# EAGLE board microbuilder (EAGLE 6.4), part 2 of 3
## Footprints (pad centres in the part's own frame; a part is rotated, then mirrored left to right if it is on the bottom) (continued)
LOWPASSFILTER0603 = smd 0.2 x 0.6: P$1 0.5,0.55; P$2 0,0.55; P$3 -0.5,0.55; P$4 -0.5,-0.55; P$5 0,-0.55; P$6 0.5,-0.55
LQFP48 = smd 1.5 x 0.25: 1 -4.3,2.75; 2 -4.3,2.25; 3 -4.3,1.75; 4 -4.3,1.25; 5 -4.3,0.75; 6 -4.3,0.25; 7 -4.3,-0.25; 8 -4.3,-0.75; 9 -4.3,-1.25; 10 -4.3,-1.75; 11 -4.3,-2.25; 12 -4.3,-2.75; 25 4.3,-2.75; 26 4.3,-2.25; 27 4.3,-1.75; 28 4.3,-1.25; 29 4.3,-0.75; 30 4.3,-0.25; 31 4.3,0.25; 32 4.3,0.75; 33 4.3,1.25; 34 4.3,1.75; 35 4.3,2.25; 36 4.3,2.75 | smd 0.25 x 1.5: 13 -2.75,-4.3; 14 -2.25,-4.3; 15 -1.75,-4.3; 16 -1.25,-4.3; 17 -0.75,-4.3; 18 -0.25,-4.3; 19 0.25,-4.3; 20 0.75,-4.3; 21 1.25,-4.3; 22 1.75,-4.3; 23 2.25,-4.3; 24 2.75,-4.3; 37 2.75,4.3; 38 2.25,4.3; 39 1.75,4.3; 40 1.25,4.3; 41 0.75,4.3; 42 0.25,4.3; 43 -0.25,4.3; 44 -0.75,4.3; 45 -1.25,4.3; 46 -1.75,4.3; 47 -2.25,4.3; 48 -2.75,4.3
LQFP64 = smd 1.55 x 0.25: 1 -5.7,3.75; 2 -5.7,3.25; 3 -5.7,2.75; 4 -5.7,2.25; 5 -5.7,1.75; 6 -5.7,1.25; 7 -5.7,0.75; 8 -5.7,0.25; 9 -5.7,-0.25; 10 -5.7,-0.75; 11 -5.7,-1.25; 12 -5.7,-1.75; 13 -5.7,-2.25; 14 -5.7,-2.75; 15 -5.7,-3.25; 16 -5.7,-3.75; 33 5.7,-3.75; 34 5.7,-3.25; 35 5.7,-2.75; 36 5.7,-2.25; 37 5.7,-1.75; 38 5.7,-1.25; 39 5.7,-0.75; 40 5.7,-0.25; 41 5.7,0.25; 42 5.7,0.75; 43 5.7,1.25; 44 5.7,1.75; 45 5.7,2.25; 46 5.7,2.75; 47 5.7,3.25; 48 5.7,3.75 | smd 0.25 x 1.55: 17 -3.75,-5.7; 18 -3.25,-5.7; 19 -2.75,-5.7; 20 -2.25,-5.7; 21 -1.75,-5.7; 22 -1.25,-5.7; 23 -0.75,-5.7; 24 -0.25,-5.7; 25 0.25,-5.7; 26 0.75,-5.7; 27 1.25,-5.7; 28 1.75,-5.7; 29 2.25,-5.7; 30 2.75,-5.7; 31 3.25,-5.7; 32 3.75,-5.7; 49 3.75,5.7; 50 3.25,5.7; 51 2.75,5.7; 52 2.25,5.7; 53 1.75,5.7; 54 1.25,5.7; 55 0.75,5.7; 56 0.25,5.7; 57 -0.25,5.7; 58 -0.75,5.7; 59 -1.25,5.7; 60 -1.75,5.7; 61 -2.25,5.7; 62 -2.75,5.7; 63 -3.25,5.7; 64 -3.75,5.7
LQFP80 = smd 1.2 x 0.254: 1 -6.725,4.75; 2 -6.725,4.25; 3 -6.725,3.75; 4 -6.725,3.25; 5 -6.725,2.75; 6 -6.725,2.25; 7 -6.725,1.75; 8 -6.725,1.25; 9 -6.725,0.75; 10 -6.725,0.25; 11 -6.725,-0.25; 12 -6.725,-0.75; 13 -6.725,-1.25; 14 -6.725,-1.75; 15 -6.725,-2.25; 16 -6.725,-2.75; 17 -6.725,-3.25; 18 -6.725,-3.75; 19 -6.725,-4.25; 20 -6.725,-4.75; 41 6.725,-4.75; 42 6.725,-4.25; 43 6.725,-3.75; 44 6.725,-3.25; 45 6.725,-2.75; 46 6.725,-2.25; 47 6.725,-1.75; 48 6.725,-1.25; 49 6.725,-0.75; 50 6.725,-0.25; 51 6.725,0.25; 52 6.725,0.75; 53 6.725,1.25; 54 6.725,1.75; 55 6.725,2.25; 56 6.725,2.75; 57 6.725,3.25; 58 6.725,3.75; 59 6.725,4.25; 60 6.725,4.75 | smd 0.254 x 1.2: 21 -4.75,-6.725; 22 -4.25,-6.725; 23 -3.75,-6.725; 24 -3.25,-6.725; 25 -2.75,-6.725; 26 -2.25,-6.725; 27 -1.75,-6.725; 28 -1.25,-6.725; 29 -0.75,-6.725; 30 -0.25,-6.725; 31 0.25,-6.725; 32 0.75,-6.725; 33 1.25,-6.725; 34 1.75,-6.725; 35 2.25,-6.725; 36 2.75,-6.725; 37 3.25,-6.725; 38 3.75,-6.725; 39 4.25,-6.725; 40 4.75,-6.725; 61 4.75,6.725; 62 4.25,6.725; 63 3.75,6.725; 64 3.25,6.725; 65 2.75,6.725; 66 2.25,6.725; 67 1.75,6.725; 68 1.25,6.725; 69 0.75,6.725; 70 0.25,6.725; 71 -0.25,6.725; 72 -0.75,6.725; 73 -1.25,6.725; 74 -1.75,6.725; 75 -2.25,6.725; 76 -2.75,6.725; 77 -3.25,6.725; 78 -3.75,6.725; 79 -4.25,6.725; 80 -4.75,6.725
LQFP100 = smd 0.27 x 1.5: 1 -6,-7.75; 2 -5.5,-7.75; 3 -5,-7.75; 4 -4.5,-7.75; 5 -4,-7.75; 6 -3.5,-7.75; 7 -3,-7.75; 8 -2.5,-7.75; 9 -2,-7.75; 10 -1.5,-7.75; 11 -1,-7.75; 12 -0.5,-7.75; 13 0,-7.75; 14 0.5,-7.75; 15 1,-7.75; 16 1.5,-7.75; 17 2,-7.75; 18 2.5,-7.75; 19 3,-7.75; 20 3.5,-7.75; 21 4,-7.75; 22 4.5,-7.75; 23 5,-7.75; 24 5.5,-7.75; 25 6,-7.75; 51 6,7.75; 52 5.5,7.75; 53 5,7.75; 54 4.5,7.75; 55 4,7.75; 56 3.5,7.75; 57 3,7.75; 58 2.5,7.75; 59 2,7.75; 60 1.5,7.75; 61 1,7.75; 62 0.5,7.75; 63 0,7.75; 64 -0.5,7.75; 65 -1,7.75; 66 -1.5,7.75; 67 -2,7.75; 68 -2.5,7.75; 69 -3,7.75; 70 -3.5,7.75; 71 -4,7.75; 72 -4.5,7.75; 73 -5,7.75; 74 -5.5,7.75; 75 -6,7.75 | smd 1.5 x 0.27: 26 7.75,-6; 27 7.75,-5.5; 28 7.75,-5; 29 7.75,-4.5; 30 7.75,-4; 31 7.75,-3.5; 32 7.75,-3; 33 7.75,-2.5; 34 7.75,-2; 35 7.75,-1.5; 36 7.75,-1; 37 7.75,-0.5; 38 7.75,0; 39 7.75,0.5; 40 7.75,1; 41 7.75,1.5; 42 7.75,2; 43 7.75,2.5; 44 7.75,3; 45 7.75,3.5; 46 7.75,4; 47 7.75,4.5; 48 7.75,5; 49 7.75,5.5; 50 7.75,6; 76 -7.75,6; 77 -7.75,5.5; 78 -7.75,5; 79 -7.75,4.5; 80 -7.75,4; 81 -7.75,3.5; 82 -7.75,3; 83 -7.75,2.5; 84 -7.75,2; 85 -7.75,1.5; 86 -7.75,1; 87 -7.75,0.5; 88 -7.75,0; 89 -7.75,-0.5; 90 -7.75,-1; 91 -7.75,-1.5; 92 -7.75,-2; 93 -7.75,-2.5; 94 -7.75,-3; 95 -7.75,-3.5; 96 -7.75,-4; 97 -7.75,-4.5; 98 -7.75,-5; 99 -7.75,-5.5; 100 -7.75,-6
LQFP144 = smd 0.27 x 1.5: 1 -8.75,-10.75; 2 -8.25,-10.75; 3 -7.75,-10.75; 4 -7.25,-10.75; 5 -6.75,-10.75; 6 -6.25,-10.75; 7 -5.75,-10.75; 8 -5.25,-10.75; 9 -4.75,-10.75; 10 -4.25,-10.75; 11 -3.75,-10.75; 12 -3.25,-10.75; 13 -2.75,-10.75; 14 -2.25,-10.75; 15 -1.75,-10.75; 16 -1.25,-10.75; 17 -0.75,-10.75; 18 -0.25,-10.75; 19 0.25,-10.75; 20 0.75,-10.75; 21 1.25,-10.75; 22 1.75,-10.75; 23 2.25,-10.75; 24 2.75,-10.75; 25 3.25,-10.75; 26 3.75,-10.75; 27 4.25,-10.75; 28 4.75,-10.75; 29 5.25,-10.75; 30 5.75,-10.75; 31 6.25,-10.75; 32 6.75,-10.75; 33 7.25,-10.75; 34 7.75,-10.75; 35 8.25,-10.75; 36 8.75,-10.75; 73 8.75,10.75; 74 8.25,10.75; 75 7.75,10.75; 76 7.25,10.75; 77 6.75,10.75; 78 6.25,10.75; 79 5.75,10.75; 80 5.25,10.75; 81 4.75,10.75; 82 4.25,10.75; 83 3.75,10.75; 84 3.25,10.75; 85 2.75,10.75; 86 2.25,10.75; 87 1.75,10.75; 88 1.25,10.75; 89 0.75,10.75; 90 0.25,10.75; 91 -0.25,10.75; 92 -0.75,10.75; 93 -1.25,10.75; 94 -1.75,10.75; 95 -2.25,10.75; 96 -2.75,10.75; 97 -3.25,10.75; 98 -3.75,10.75; 99 -4.25,10.75; 100 -4.75,10.75; 101 -5.25,10.75; 102 -5.75,10.75; 103 -6.25,10.75; 104 -6.75,10.75; 105 -7.25,10.75; 106 -7.75,10.75; 107 -8.25,10.75; 108 -8.75,10.75 | smd 1.5 x 0.27: 37 10.75,-8.75; 38 10.75,-8.25; 39 10.75,-7.75; 40 10.75,-7.25; 41 10.75,-6.75; 42 10.75,-6.25; 43 10.75,-5.75; 44 10.75,-5.25; 45 10.75,-4.75; 46 10.75,-4.25; 47 10.75,-3.75; 48 10.75,-3.25; 49 10.75,-2.75; 50 10.75,-2.25; 51 10.75,-1.75; 52 10.75,-1.25; 53 10.75,-0.75; 54 10.75,-0.25; 55 10.75,0.25; 56 10.75,0.75; 57 10.75,1.25; 58 10.75,1.75; 59 10.75,2.25; 60 10.75,2.75; 61 10.75,3.25; 62 10.75,3.75; 63 10.75,4.25; 64 10.75,4.75; 65 10.75,5.25; 66 10.75,5.75; 67 10.75,6.25; 68 10.75,6.75; 69 10.75,7.25; 70 10.75,7.75; 71 10.75,8.25; 72 10.75,8.75; 109 -10.75,8.75; 110 -10.75,8.25; 111 -10.75,7.75; 112 -10.75,7.25; 113 -10.75,6.75; 114 -10.75,6.25; 115 -10.75,5.75; 116 -10.75,5.25; 117 -10.75,4.75; 118 -10.75,4.25; 119 -10.75,3.75; 120 -10.75,3.25; 121 -10.75,2.75; 122 -10.75,2.25; 123 -10.75,1.75; 124 -10.75,1.25; 125 -10.75,0.75; 126 -10.75,0.25; 127 -10.75,-0.25; 128 -10.75,-0.75; 129 -10.75,-1.25; 130 -10.75,-1.75; 131 -10.75,-2.25; 132 -10.75,-2.75; 133 -10.75,-3.25; 134 -10.75,-3.75; 135 -10.75,-4.25; 136 -10.75,-4.75; 137 -10.75,-5.25; 138 -10.75,-5.75; 139 -10.75,-6.25; 140 -10.75,-6.75; 141 -10.75,-7.25; 142 -10.75,-7.75; 143 -10.75,-8.25; 144 -10.75,-8.75
LQFP208 = smd 1.4 x 0.29: 1 -15.3,12.75; 2 -15.3,12.25; 3 -15.3,11.75; 4 -15.3,11.25; 5 -15.3,10.75; 6 -15.3,10.25; 7 -15.3,9.75; 8 -15.3,9.25; 9 -15.3,8.75; 10 -15.3,8.25; 11 -15.3,7.75; 12 -15.3,7.25; 13 -15.3,6.75; 14 -15.3,6.25; 15 -15.3,5.75; 16 -15.3,5.25; 17 -15.3,4.75; 18 -15.3,4.25; 19 -15.3,3.75; 20 -15.3,3.25; 21 -15.3,2.75; 22 -15.3,2.25; 23 -15.3,1.75; 24 -15.3,1.25; 25 -15.3,0.75; 26 -15.3,0.25; 27 -15.3,-0.25; 28 -15.3,-0.75; 29 -15.3,-1.25; 30 -15.3,-1.75; 31 -15.3,-2.25; 32 -15.3,-2.75; 33 -15.3,-3.25; 34 -15.3,-3.75; 35 -15.3,-4.25; 36 -15.3,-4.75; 37 -15.3,-5.25; 38 -15.3,-5.75; 39 -15.3,-6.25; 40 -15.3,-6.75; 41 -15.3,-7.25; 42 -15.3,-7.75; 43 -15.3,-8.25; 44 -15.3,-8.75; 45 -15.3,-9.25; 46 -15.3,-9.75; 47 -15.3,-10.25; 48 -15.3,-10.75; 49 -15.3,-11.25; 50 -15.3,-11.75; 51 -15.3,-12.25; 52 -15.3,-12.75; 105 15.3,-12.75; 106 15.3,-12.25; 107 15.3,-11.75; 108 15.3,-11.25; 109 15.3,-10.75; 110 15.3,-10.25; 111 15.3,-9.75; 112 15.3,-9.25; 113 15.3,-8.75; 114 15.3,-8.25; 115 15.3,-7.75; 116 15.3,-7.25; 117 15.3,-6.75; 118 15.3,-6.25; 119 15.3,-5.75; 120 15.3,-5.25; 121 15.3,-4.75; 122 15.3,-4.25; 123 15.3,-3.75; 124 15.3,-3.25; 125 15.3,-2.75; 126 15.3,-2.25; 127 15.3,-1.75; 128 15.3,-1.25; 129 15.3,-0.75; 130 15.3,-0.25; 131 15.3,0.25; 132 15.3,0.75; 133 15.3,1.25; 134 15.3,1.75; 135 15.3,2.25; 136 15.3,2.75; 137 15.3,3.25; 138 15.3,3.75; 139 15.3,4.25; 140 15.3,4.75; 141 15.3,5.25; 142 15.3,5.75; 143 15.3,6.25; 144 15.3,6.75; 145 15.3,7.25; 146 15.3,7.75; 147 15.3,8.25; 148 15.3,8.75; 149 15.3,9.25; 150 15.3,9.75; 151 15.3,10.25; 152 15.3,10.75; 153 15.3,11.25; 154 15.3,11.75; 155 15.3,12.25; 156 15.3,12.75 | smd 0.29 x 1.4: 53 -12.75,-15.3; 54 -12.25,-15.3; 55 -11.75,-15.3; 56 -11.25,-15.3; 57 -10.75,-15.3; 58 -10.25,-15.3; 59 -9.75,-15.3; 60 -9.25,-15.3; 61 -8.75,-15.3; 62 -8.25,-15.3; 63 -7.75,-15.3; 64 -7.25,-15.3; 65 -6.75,-15.3; 66 -6.25,-15.3; 67 -5.75,-15.3; 68 -5.25,-15.3; 69 -4.75,-15.3; 70 -4.25,-15.3; 71 -3.75,-15.3; 72 -3.25,-15.3; 73 -2.75,-15.3; 74 -2.25,-15.3; 75 -1.75,-15.3; 76 -1.25,-15.3; 77 -0.75,-15.3; 78 -0.25,-15.3; 79 0.25,-15.3; 80 0.75,-15.3; 81 1.25,-15.3; 82 1.75,-15.3; 83 2.25,-15.3; 84 2.75,-15.3; 85 3.25,-15.3; 86 3.75,-15.3; 87 4.25,-15.3; 88 4.75,-15.3; 89 5.25,-15.3; 90 5.75,-15.3; 91 6.25,-15.3; 92 6.75,-15.3; 93 7.25,-15.3; 94 7.75,-15.3; 95 8.25,-15.3; 96 8.75,-15.3; 97 9.25,-15.3; 98 9.75,-15.3; 99 10.25,-15.3; 100 10.75,-15.3; 101 11.25,-15.3; 102 11.75,-15.3; 103 12.25,-15.3; 104 12.75,-15.3; 157 12.75,15.3; 158 12.25,15.3; 159 11.75,15.3; 160 11.25,15.3; 161 10.75,15.3; 162 10.25,15.3; 163 9.75,15.3; 164 9.25,15.3; 165 8.75,15.3; 166 8.25,15.3; 167 7.75,15.3; 168 7.25,15.3; 169 6.75,15.3; 170 6.25,15.3; 171 5.75,15.3; 172 5.25,15.3; 173 4.75,15.3; 174 4.25,15.3; 175 3.75,15.3; 176 3.25,15.3; 177 2.75,15.3; 178 2.25,15.3; 179 1.75,15.3; 180 1.25,15.3; 181 0.75,15.3; 182 0.25,15.3; 183 -0.25,15.3; 184 -0.75,15.3; 185 -1.25,15.3; 186 -1.75,15.3; 187 -2.25,15.3; 188 -2.75,15.3; 189 -3.25,15.3; 190 -3.75,15.3; 191 -4.25,15.3; 192 -4.75,15.3; 193 -5.25,15.3; 194 -5.75,15.3; 195 -6.25,15.3; 196 -6.75,15.3; 197 -7.25,15.3; 198 -7.75,15.3; 199 -8.25,15.3; 200 -8.75,15.3; 201 -9.25,15.3; 202 -9.75,15.3; 203 -10.25,15.3; 204 -10.75,15.3; 205 -11.25,15.3; 206 -11.75,15.3; 207 -12.25,15.3; 208 -12.75,15.3
MICROSD = smd 0.7 x 1.5: 1 9,-10.64; 2 7.9,-10.24; 3 6.8,-10.64; 4 5.7,-11.04; 5 4.6,-10.64; 6 3.5,-11.04; 7 2.4,-10.64; 8 1.3,-10.64 | smd 1.8 x 1.4: CD1 2,-0.44; CD2 8,-0.44 | smd 1.4 x 1.9: MT1 0.4,-13.54; MT2 13.6,-14.44
MINIMOLD6 = smd 0.26 x 0.65: P$1 -0.5,-0.65; P$2 0,-0.65; P$3 0.5,-0.65; P$4 0.5,0.65; P$5 0,0.65; P$6 -0.5,0.65
MOLEX20_RIGHTANGLE = smd 1 x 4: 1 11.43,0; 3 8.89,0; 5 6.35,0; 7 3.81,0; 9 1.27,0; 11 -1.27,0; 13 -3.81,0; 15 -6.35,0; 17 -8.89,0; 19 -11.43,0 | smd 1 x 4 bottom: 2 11.43,0; 4 8.89,0; 6 6.35,0; 8 3.81,0; 10 1.27,0; 12 -1.27,0; 14 -3.81,0; 16 -6.35,0; 18 -8.89,0; 20 -11.43,0
MOUNTINGHOLE_1.0_PLATED = drill 1 pad 3: P$1 0,0
MOUNTINGHOLE_2.0_PLATED = drill 2.2 pad 3: P$1 0,0
MOUNTINGHOLE_2.5_PLATED = drill 2.5 pad 3.2: P$1 0,0
MOUNTINGHOLE_2.5_PLATED_THICK = drill 2.5 pad 4: P$1 0,0
MOUNTINGHOLE_2.8 = hole 2.8: 0,0
MOUNTINGHOLE_3.0 = hole 3: 0,0
MOUNTINGHOLE_3.0_PLATED = drill 3 pad 6.452: P$1 0,0
MOUNTINGHOLE_3.0_PLATEDTHIN = drill 3 pad 3.6: P$1 0,0
MOUNTINGHOLE_3.2 = hole 3.2: 0,0
MSOP8_0.65MM = smd 0.4 x 1.4: 1 -0.975,-2.2; 2 -0.325,-2.2; 3 0.325,-2.2; 4 0.975,-2.2; 5 0.975,2.2; 6 0.325,2.2; 7 -0.325,2.2; 8 -0.975,2.2
MSOP10 = smd 0.25 x 1: 1 -1,-2.113; 2 -0.5,-2.113; 3 0,-2.113; 4 0.5,-2.113; 5 1,-2.113; 6 1,2.113; 7 0.5,2.113; 8 0,2.113; 9 -0.5,2.113; 10 -1,2.113
OSC_3.2X2.5MM = smd 1.4 x 1.2: 1 -1.1,-0.8; 2 1.1,-0.8; 3 1.1,0.8; 4 -1.1,0.8
OSC_7X5MM = smd 1.8 x 2: 1 -2.54,-2.1; 2 2.54,-2.1; 3 2.54,2.1; 4 -2.54,2.1
PAD-1.5X2.0 = smd 1.5 x 2: P$1 0,0
PANASONIC_C = smd 2.6 x 1.4: + 2.05,0; - -2.05,0
PANASONIC_D = smd 3.556 x 1.4: + 2.654,0; - -2.654,0
PSP_BACKLIGHTCON = smd 0.28 x 1.4: NC1 -0.25,0; NC2 0.25,0; VLED+ 0.75,0; VLED- -0.75,0 | smd 2.667 x 1.27: P$1 -2.54,-1.27; P$2 2.54,-1.27
PSP_TSCON = smd 0.6 x 2.3: X1 1.5,1.15; X2 -0.5,1.15; Y1 -1.5,1.15; Y2 0.5,1.15
PTC1210 = smd 1 x 3.2: P$1 -1.5,0; P$2 1.5,0
PTC1812 = smd 1.5 x 3.7: P$1 -2.1,0; P$2 2.1,0
PUSHBUTTON_SMD_SJ = smd 2 x 2: P$1 3,0; P$2 -3,0
QFN16_3MM = smd 0.8 x 0.28: P$1 -1.5,0.75; P$2 -1.5,0.25; P$3 -1.5,-0.25; P$4 -1.5,-0.75; P$9 1.5,-0.75; P$10 1.5,-0.25; P$11 1.5,0.25; P$12 1.5,0.75 | smd 0.28 x 0.8: P$5 -0.75,-1.5; P$6 -0.25,-1.5; P$7 0.25,-1.5; P$8 0.75,-1.5; P$13 0.75,1.5; P$14 0.25,1.5; P$15 -0.25,1.5; P$16 -0.75,1.5 | smd 1.5 x 1.5: THERMAL 0,0
QFN20_3MM = smd 0.7 x 0.2: 1 -1.4,0.8; 2 -1.4,0.4; 3 -1.4,0; 4 -1.4,-0.4; 5 -1.4,-0.8; 11 1.4,-0.8; 12 1.4,-0.4; 13 1.4,0; 14 1.4,0.4; 15 1.4,0.8 | smd 0.2 x 0.7: 6 -0.8,-1.4; 7 -0.4,-1.4; 8 0,-1.4; 9 0.4,-1.4; 10 0.8,-1.4; 16 0.8,1.4; 17 0.4,1.4; 18 0,1.4; 19 -0.4,1.4; 20 -0.8,1.4 | smd 1.6 x 1.6: 21 0,0
QFN20_4MM = smd 0.73 x 0.28: P$1 -1.965,1; P$2 -1.965,0.5; P$3 -1.965,0; P$4 -1.965,-0.5; P$5 -1.965,-1; P$11 1.965,-1; P$12 1.965,-0.5; P$13 1.965,0; P$14 1.965,0.5; P$15 1.965,1 | smd 0.28 x 0.73: P$6 -1,-1.965; P$7 -0.5,-1.965; P$8 0,-1.965; P$9 0.5,-1.965; P$10 1,-1.965; P$16 1,1.965; P$17 0.5,1.965; P$18 0,1.965; P$19 -0.5,1.965; P$20 -1,1.965 | smd 2.5 x 2.5: P$21 0,0
QFN24_4MM = smd 0.8 x 0.28: 1 -2,1.25; 2 -2,0.75; 3 -2,0.25; 4 -2,-0.25; 5 -2,-0.75; 6 -2,-1.25; 13 2,-1.25; 14 2,-0.75; 15 2,-0.25; 16 2,0.25; 17 2,0.75; 18 2,1.25 | smd 0.28 x 0.8: 7 -1.25,-2; 8 -0.75,-2; 9 -0.25,-2; 10 0.25,-2; 11 0.75,-2; 12 1.25,-2; 19 1.25,2; 20 0.75,2; 21 0.25,2; 22 -0.25,2; 23 -0.75,2; 24 -1.25,2 | smd 1.778 x 1.778: THERM 0,0
QFN28_5MM = smd 1.15 x 0.27: 1 -2.4,1.5; 2 -2.4,1; 3 -2.4,0.5; 4 -2.4,0; 5 -2.4,-0.5; 6 -2.4,-1; 7 -2.4,-1.5; 15 2.4,-1.5; 16 2.4,-1; 17 2.4,-0.5; 18 2.4,0; 19 2.4,0.5; 20 2.4,1; 21 2.4,1.5 | smd 0.27 x 1.15: 8 -1.5,-2.4; 9 -1,-2.4; 10 -0.5,-2.4; 11 0,-2.4; 12 0.5,-2.4; 13 1,-2.4; 14 1.5,-2.4; 22 1.5,2.4; 23 1,2.4; 24 0.5,2.4; 25 0,2.4; 26 -0.5,2.4; 27 -1,2.4; 28 -1.5,2.4 | smd 3.15 x 3.15: THERMAL 0,0
QFN32_5MM = smd 0.8 x 0.25: 1 -2.5,1.75; 2 -2.5,1.25; 3 -2.5,0.75; 4 -2.5,0.25; 5 -2.5,-0.25; 6 -2.5,-0.75; 7 -2.5,-1.25; 8 -2.5,-1.75; 17 2.5,-1.75; 18 2.5,-1.25; 19 2.5,-0.75; 20 2.5,-0.25; 21 2.5,0.25; 22 2.5,0.75; 23 2.5,1.25; 24 2.5,1.75 | smd 0.25 x 0.8: 9 -1.75,-2.5; 10 -1.25,-2.5; 11 -0.75,-2.5; 12 -0.25,-2.5; 13 0.25,-2.5; 14 0.75,-2.5; 15 1.25,-2.5; 16 1.75,-2.5; 25 1.75,2.5; 26 1.25,2.5; 27 0.75,2.5; 28 0.25,2.5; 29 -0.25,2.5; 30 -0.75,2.5; 31 -1.25,2.5; 32 -1.75,2.5 | smd 3.5 x 3.5: 33 0,0
QSOP24_0.635MM = smd 0.3 x 1.7: 1 -3.493,-2.935; 2 -2.857,-2.935; 3 -2.223,-2.935; 4 -1.587,-2.935; 5 -0.953,-2.935; 6 -0.318,-2.935; 7 0.318,-2.935; 8 0.953,-2.935; 9 1.587,-2.935; 10 2.223,-2.935; 11 2.857,-2.935; 12 3.493,-2.935; 13 3.493,2.935; 14 2.857,2.935; 15 2.223,2.935; 16 1.587,2.935; 17 0.953,2.935; 18 0.318,2.935; 19 -0.318,2.935; 20 -0.953,2.935; 21 -1.587,2.935; 22 -2.223,2.935; 23 -2.857,2.935; 24 -3.493,2.935
RASBERRYPI_IDC = drill 1 pad 1.676 square: 1 -1.27,15.24 | drill 1 pad 1.676: 2 1.27,15.24; 3 -1.27,12.7; 4 1.27,12.7; 5 -1.27,10.16; 6 1.27,10.16; 7 -1.27,7.62; 8 1.27,7.62; 9 -1.27,5.08; 10 1.27,5.08; 11 -1.27,2.54; 12 1.27,2.54; 13 -1.27,0; 14 1.27,0; 15 -1.27,-2.54; 16 1.27,-2.54; 17 -1.27,-5.08; 18 1.27,-5.08; 19 -1.27,-7.62; 20 1.27,-7.62; 21 -1.27,-10.16; 22 1.27,-10.16; 23 -1.27,-12.7; 24 1.27,-12.7; 25 -1.27,-15.24; 26 1.27,-15.24
RASBERRYPI_SHIELD = drill 1 pad 1.676 square: 1 51.308,82.55 | drill 1 pad 1.676: 2 53.848,82.55; 3 51.308,80.01; 4 53.848,80.01; 5 51.308,77.47; 6 53.848,77.47; 7 51.308,74.93; 8 53.848,74.93; 9 51.308,72.39; 10 53.848,72.39; 11 51.308,69.85; 12 53.848,69.85; 13 51.308,67.31; 14 53.848,67.31; 15 51.308,64.77; 16 53.848,64.77; 17 51.308,62.23; 18 53.848,62.23; 19 51.308,59.69; 20 53.848,59.69; 21 51.308,57.15; 22 53.848,57.15; 23 51.308,54.61; 24 53.848,54.61; 25 51.308,52.07; 26 53.848,52.07
RESPACK_4X0603 = smd 0.65 x 0.8: 1 -1.3,-0.75; 4 1.3,-0.75; 5 1.3,0.75; 8 -1.3,0.75 | smd 0.5 x 0.8: 2 -0.4,-0.75; 3 0.4,-0.75; 6 0.4,0.75; 7 -0.4,0.75
RGBLED_PLCC4 = smd 1.1 x 1: 1 -1.4,0.6; 2 -1.4,-0.6; 3 1.4,-0.6; 4 1.4,0.6
RGBLED_PLCC6 = smd 1 x 2: 1 -1.6,-2.158; 2 0,-2.158; 3 1.6,-2.158; 4 1.6,2.108; 5 0,2.108; 6 -1.6,2.108
RJ45PTH = drill 0.9: 1 3.57,2.54; 2 2.55,4.32; 3 1.53,2.54; 4 0.51,4.32; 5 -0.51,2.54; 6 -1.53,4.32; 7 -2.55,2.54; 8 -3.57,4.32; 9 -6.86,9.18; 10 -4.57,9.18; 11 4.57,9.18; 12 6.86,9.18 | drill 1.6: P$11 -8.13,3.43; P$12 8.13,3.43 | hole 3.2: -6.35,0; 6.35,0
RJ45SMT = smd 0.61 x 3.05: 1 3.57,9.98; 2 2.55,9.98; 3 1.53,9.98; 4 0.51,9.98; 5 -0.51,9.98; 6 -1.53,9.98; 7 -2.55,9.98; 8 -3.57,9.98; 9 -6.975,10.8; 10 -5.705,10.8; 11 5.705,10.8; 12 6.975,10.8 | smd 2 x 3.05: P$13 8.66,0; P$14 -8.89,0 | hole 3.25: -6.35,0; 6.35,0
RJ45_PULSEJACK = drill 0.9: 1 4.445,-6.35; 2 3.175,-8.89; 3 1.905,-6.35; 4 0.635,-8.89; 5 -0.635,-6.35; 6 -1.905,-8.89; 7 -3.175,-6.35; 8 -4.445,-8.89 | drill 1: 9 6.325,4.9; 10 3.785,3.38; 11 -3.785,4.9; 12 -6.325,3.38 | drill 1.6: P$5 -7.875,-3.05; P$6 7.875,-3.05 | hole 3.2: -5.715,0; 5.715,0
S6B33B6_1.5IN_LCD = smd 0.5 x 3: P$1 -12.8,-6.25; P$2 -12,-6.25; P$3 -11.2,-6.25; P$4 -10.4,-6.25; P$5 -9.6,-6.25; P$6 -8.8,-6.25; P$7 -8,-6.25; P$8 -7.2,-6.25; P$9 -6.4,-6.25; P$10 -5.6,-6.25; P$11 -4.8,-6.25; P$12 -4,-6.25; P$13 -3.2,-6.25; P$14 -2.4,-6.25; P$15 -1.6,-6.25; P$16 -0.8,-6.25; P$17 0,-6.25; P$18 0.8,-6.25; P$19 1.6,-6.25; P$20 2.4,-6.25; P$21 3.2,-6.25; P$22 4,-6.25; P$23 4.8,-6.25; P$24 5.6,-6.25; P$25 6.4,-6.25; P$26 7.2,-6.25; P$27 8,-6.25; P$28 8.8,-6.25; P$29 9.6,-6.25; P$30 10.4,-6.25; P$31 11.2,-6.25; P$32 12,-6.25; P$33 12.8,-6.25 | hole 1: 12.8,-9.8; -12.8,-9.8
SC70-6L = smd 0.35 x 0.8: 1 -0.65,-0.85; 2 0,-0.85; 3 0.65,-0.85; 4 0.65,0.85; 5 0,0.85; 6 -0.65,0.85
SDCARD_PCBCARRIER_DIM = smd 1.4 x 3.4: P$1 -6.875,0; P$2 -4.375,0; P$5 3.125,0; P$6 5.625,0; P$9 -9.375,-2.3 | smd 1.4 x 3.6: P$3 -1.875,0.1; P$4 0.625,0.1 | smd 1.1 x 3.4: P$7 8.05,0 | smd 0.9 x 3.4: P$8 9.75,0
SDCARD_PCBCARRIER_DOCU = smd 1.4 x 3.4: P$1 -6.875,0; P$2 -4.375,0; P$5 3.125,0; P$6 5.625,0; P$9 -9.375,-2.3 | smd 1.4 x 3.6: P$3 -1.875,0.1; P$4 0.625,0.1 | smd 1.1 x 3.4: P$7 8.05,0 | smd 0.9 x 3.4: P$8 9.75,0
SDCARD_SMT_4U06132 = smd 1 x 2.008: 1 6.88,11.254; 2 4.38,11.254; 3 1.88,11.254; 4 -0.62,11.254; 5 -3.12,11.254; 6 -5.62,11.254; 7 -8.12,11.254; 9 9.38,11.254 | smd 0.6 x 2.008: 8 -9.845,11.254; CD -11.045,11.254; WP -12.245,11.254 | smd 1.6 x 2.8: GND -14.1,-12.35; NC1 -14.1,9.15; NC2 11.631,9.15; NC3 13.6,-12.35 | hole 1.6: 9.5,8.2 | hole 1.1: -11.5,8.2
SDCARD_SMT_4U19646 = smd 1.05 x 1.56: CD 1.02,15.47; P$1 6.77,15.47; P$2 4.27,15.47; P$3 2.52,15.47; P$4 -0.73,15.47; P$5 -3.23,15.47; P$6 -5.73,15.47; P$7 -8.15,15.47; P$8 -9.85,15.47; P$9 9.27,15.47; WP -13.2,15.47 | smd 1.2 x 2: GND@1 14.8,-5.6; GND@2 -14.8,-5.6 | hole 1.8: -12.1,-8.9; 12.1,-8.9
SEGMENT-BL-Q56C43 = drill 0.8 pad 1.778: P$1 -7.62,-7.62; P$2 -5.08,-7.62; P$3 -2.54,-7.62; P$4 0,-7.62; P$5 2.54,-7.62; P$6 5.08,-7.62; P$7 7.62,-7.62; P$8 7.62,7.62; P$9 5.08,7.62; P$10 2.54,7.62; P$11 0,7.62; P$12 -2.54,7.62; P$13 -5.08,7.62; P$14 -7.62,7.62
SEGMENT_BICOL_BL-AR12Z3010 = drill 0.8 pad 1.676: 1 -3.6,7.57; 2 -3.6,5.03; 3 -3.6,2.49; 4 -3.6,-0.05; 5 -3.6,-2.59; 6 -3.6,-5.13; 7 -3.6,-7.67; 8 3.6,-7.57; 9 3.6,-5.03; 10 3.6,-2.49; 11 3.6,0.05; 12 3.6,2.59; 13 3.6,5.13; 14 3.6,7.67
SEGMENT_BICOL_BL-M12A883XX = drill 0.8 pad 1.676: 1 -13.97,-12; 2 -11.43,-12; 3 -8.89,-12; 4 -6.35,-12; 5 -3.81,-12; 6 -1.27,-12; 7 1.27,-12; 8 3.81,-12; 9 6.35,-12; 10 8.89,-12; 11 11.43,-12; 12 13.97,-12; 13 13.97,12; 14 11.43,12; 15 8.89,12; 16 6.35,12; 17 3.81,12; 18 1.27,12; 19 -1.27,12; 20 -3.81,12; 21 -6.35,12; 22 -8.89,12; 23 -11.43,12; 24 -13.97,12
SEGMENT_BL-M07C881UR = drill 0.8 pad 1.676: 1 -8.75,-7.5; 2 -6.25,-7.5; 3 -3.75,-7.5; 4 -1.25,-7.5; 5 1.25,-7.5; 6 3.75,-7.5; 7 6.25,-7.5; 8 8.75,-7.5; 9 8.75,7.5; 10 6.25,7.5; 11 3.75,7.5; 12 1.25,7.5; 13 -1.25,7.5; 14 -3.75,7.5; 15 -6.25,7.5; 16 -8.75,7.5
SEGMENT_BL-M12A881UR = drill 0.8 pad 1.676: 1 -8.89,-12; 2 -6.35,-12; 3 -3.81,-12; 4 -1.27,-12; 5 1.27,-12; 6 3.81,-12; 7 6.35,-12; 8 8.89,-12; 9 8.89,12; 10 6.35,12; 11 3.81,12; 12 1.27,12; 13 -1.27,12; 14 -3.81,12; 15 -6.35,12; 16 -8.89,12
SEGMENT_BL-M12A883 = drill 0.8 pad 1.676: 1 -8.89,-12; 2 -6.35,-12; 3 -3.81,-12; 4 -1.27,-12; 5 1.27,-12; 6 3.81,-12; 7 6.35,-12; 8 8.89,-12; 9 8.89,12; 10 6.35,12; 11 3.81,12; 12 1.27,12; 13 -1.27,12; 14 -3.81,12; 15 -6.35,12; 16 -8.89,12
SEGMENT_BL-Q39A-42 = drill 0.8: P$1 -8.89,-5.08; P$2 -6.35,-5.08; P$3 -3.81,-5.08; P$4 -1.27,-5.08; P$5 1.27,-5.08; P$6 3.81,-5.08; P$7 6.35,-5.08; P$8 8.89,-5.08; P$9 8.89,5.08; P$10 6.35,5.08; P$11 3.81,5.08; P$12 1.27,5.08; P$13 -1.27,5.08; P$14 -3.81,5.08; P$15 -6.35,5.08; P$16 -8.89,5.08
SEGMENT_STARBURST_BL-S80A-13 = drill 0.8 pad 1.676: 1 -7.62,10.16; 2 -7.62,7.62; 3 -7.62,5.08; 4 -7.62,2.54; 5 -7.62,0; 6 -7.62,-2.54; 7 -7.62,-5.08; 8 -7.62,-7.62; 9 -7.62,-10.16; 10 7.62,-10.16; 11 7.62,-7.62; 12 7.62,-5.08; 13 7.62,-2.54; 14 7.62,0; 15 7.62,2.54; 16 7.62,5.08; 17 7.62,7.62; 18 7.62,10.16
SEGMENT_STARBURST_BL-S230B-12 = drill 0.8 pad 1.676: 1 -11.43,-30.1; 2 -8.89,-30.1; 3 -6.35,-30.1; 4 -3.81,-30.1; 5 -1.27,-30.1; 6 1.27,-30.1; 7 3.81,-30.1; 8 6.35,-30.1; 9 8.89,-30.1; 10 11.43,-30.1; 11 11.43,30.1; 12 8.89,30.1; 13 6.35,30.1; 14 3.81,30.1; 15 1.27,30.1; 16 -1.27,30.1; 17 -3.81,30.1; 18 -6.35,30.1; 19 -8.89,30.1; 20 -11.43,30.1
SI473X_SSOP = smd 1.55 x 0.35: P$1 -2.625,3.493; P$2 -2.625,2.857; P$3 -2.625,2.223; P$4 -2.625,1.587; P$5 -2.625,0.953; P$6 -2.625,0.318; P$7 -2.625,-0.318; P$8 -2.625,-0.953; P$9 -2.625,-1.587; P$10 -2.625,-2.223; P$11 -2.625,-2.857; P$12 -2.625,-3.493; P$13 2.625,-3.493; P$14 2.625,-2.857; P$15 2.625,-2.223; P$16 2.625,-1.587; P$17 2.625,-0.953; P$18 2.625,-0.318; P$19 2.625,0.318; P$20 2.625,0.953; P$21 2.625,1.587; P$22 2.625,2.223; P$23 2.625,2.857; P$24 2.625,3.493
SIM900B_SMT = smd 0.25 x 1.35: 1 -7.25,-1.475; 2 -7.25,1.475; 3 -6.75,-1.475; 4 -6.75,1.475; 5 -6.25,-1.475; 6 -6.25,1.475; 7 -5.75,-1.475; 8 -5.75,1.475; 9 -5.25,-1.475; 10 -5.25,1.475; 11 -4.75,-1.475; 12 -4.75,1.475; 13 -4.25,-1.475; 14 -4.25,1.475; 15 -3.75,-1.475; 16 -3.75,1.475; 17 -3.25,-1.475; 18 -3.25,1.475; 19 -2.75,-1.475; 20 -2.75,1.475; 21 -2.25,-1.475; 22 -2.25,1.475; 23 -1.75,-1.475; 24 -1.75,1.475; 25 -1.25,-1.475; 26 -1.25,1.475; 27 -0.75,-1.475; 28 -0.75,1.475; 29 -0.25,-1.475; 30 -0.25,1.475; 31 0.25,-1.475; 32 0.25,1.475; 33 0.75,-1.475; 34 0.75,1.475; 35 1.25,-1.475; 36 1.25,1.475; 37 1.75,-1.475; 38 1.75,1.475; 39 2.25,-1.475; 40 2.25,1.475; 41 2.75,-1.475; 42 2.75,1.475; 43 3.25,-1.475; 44 3.25,1.475; 45 3.75,-1.475; 46 3.75,1.475; 47 4.25,-1.475; 48 4.25,1.475; 49 4.75,-1.475; 50 4.75,1.475; 51 5.25,-1.475; 52 5.25,1.475; 53 5.75,-1.475; 54 5.75,1.475; 55 6.25,-1.475; 56 6.25,1.475; 57 6.75,-1.475; 58 6.75,1.475; 59 7.25,-1.475; 60 7.25,1.475 | drill 1.5 pad 2.54: P$1 -6.63,29.25; P$2 8.09,16.86; P$3 -30.89,9.41; P$4 -14.53,-2.72
SIM900_SMT = smd 2 x 0.6: P$1 -12.4,8; P$2 -12.4,7; P$3 -12.4,6; P$4 -12.4,5; P$5 -12.4,4; P$6 -12.4,3; P$7 -12.4,2; P$8 -12.4,1; P$9 -12.4,0; P$10 -12.4,-1; P$11 -12.4,-2; P$12 -12.4,-3; P$13 -12.4,-4; P$14 -12.4,-5; P$15 -12.4,-6; P$16 -12.4,-7; P$17 -12.4,-8; P$35 12.4,-8; P$36 12.4,-7; P$37 12.4,-6; P$38 12.4,-5; P$39 12.4,-4; P$40 12.4,-3; P$41 12.4,-2; P$42 12.4,-1; P$43 12.4,0; P$44 12.4,1; P$45 12.4,2; P$46 12.4,3; P$47 12.4,4; P$48 12.4,5; P$49 12.4,6; P$50 12.4,7; P$51 12.4,8 | smd 0.6 x 2: P$18 -8,-12.4; P$19 -7,-12.4; P$20 -6,-12.4; P$21 -5,-12.4; P$22 -4,-12.4; P$23 -3,-12.4; P$24 -2,-12.4; P$25 -1,-12.4; P$26 0,-12.4; P$27 1,-12.4; P$28 2,-12.4; P$29 3,-12.4; P$30 4,-12.4; P$31 5,-12.4; P$32 6,-12.4; P$33 7,-12.4; P$34 8,-12.4; P$52 8,12.4; P$53 7,12.4; P$54 6,12.4; P$55 5,12.4; P$56 4,12.4; P$57 3,12.4; P$58 2,12.4; P$59 1,12.4; P$60 0,12.4; P$61 -1,12.4; P$62 -2,12.4; P$63 -3,12.4; P$64 -4,12.4; P$65 -5,12.4; P$66 -6,12.4; P$67 -7,12.4; P$68 -8,12.4
SIM908 = smd 1.8 x 0.6: P$1 -15,9.5; P$2 -15,8.5; P$3 -15,7.5; P$4 -15,6.5; P$5 -15,5.5; P$6 -15,4.5; P$7 -15,3.5; P$8 -15,2.5; P$9 -15,1.5; P$10 -15,0.5; P$11 -15,-0.5; P$12 -15,-1.5; P$13 -15,-2.5; P$14 -15,-3.5; P$15 -15,-4.5; P$16 -15,-5.5; P$17 -15,-6.5; P$18 -15,-7.5; P$19 -15,-8.5; P$20 -15,-9.5; P$41 15,-9.5; P$42 15,-8.5; P$43 15,-7.5; P$44 15,-6.5; P$45 15,-5.5; P$46 15,-4.5; P$47 15,-3.5; P$48 15,-2.5; P$49 15,-1.5; P$50 15,-0.5; P$51 15,0.5; P$52 15,1.5; P$53 15,2.5; P$54 15,3.5; P$55 15,4.5; P$56 15,5.5; P$57 15,6.5; P$58 15,7.5; P$59 15,8.5; P$60 15,9.5 | smd 0.6 x 1.8: P$21 -9.5,-15; P$22 -8.5,-15; P$23 -7.5,-15; P$24 -6.5,-15; P$25 -5.5,-15; P$26 -4.5,-15; P$27 -3.5,-15; P$28 -2.5,-15; P$29 -1.5,-15; P$30 -0.5,-15; P$31 0.5,-15; P$32 1.5,-15; P$33 2.5,-15; P$34 3.5,-15; P$35 4.5,-15; P$36 5.5,-15; P$37 6.5,-15; P$38 7.5,-15; P$39 8.5,-15; P$40 9.5,-15; P$61 9.5,15; P$62 8.5,15; P$63 7.5,15; P$64 6.5,15; P$65 5.5,15; P$66 4.5,15; P$67 3.5,15; P$68 2.5,15; P$69 1.5,15; P$70 0.5,15; P$71 -0.5,15; P$72 -1.5,15; P$73 -2.5,15; P$74 -3.5,15; P$75 -4.5,15; P$76 -5.5,15; P$77 -6.5,15; P$78 -7.5,15; P$79 -8.5,15; P$80 -9.5,15
SIM_5002 = smd 2.54 x 1.27: 1 0.904,0.574; 2 0.904,3.114; 3 0.904,5.654; 5 26.299,0.594; 6 26.299,3.134; 7 26.299,5.674 | hole 1.7: 21.8,-1.6 | hole 1.2: 6,10.4
SMA90_DIP = drill 1.5 pad 2.54: ANTENNA 0,0 | drill 1.6 pad 2.54: GND1 -2.54,2.54; GND2 2.54,2.54; GND3 -2.54,-2.54; GND4 2.54,-2.54
SMADIODE = smd 2.54 x 2.54: A 2.349,0; C -2.349,0
SMB_DIP = drill 1.5 pad 2.54: ANTENNA 0,0 | drill 1.6 pad 2.54: GND1 -2.54,2.54; GND2 2.54,2.54; GND3 -2.54,-2.54; GND4 2.54,-2.54
SOCKET_LBGA256_8117-256-4E-01 = drill 0.43 pad 0.7 octagon: A1 7.5,7.5; A2 7.5,6.5; A3 7.5,5.5; A4 7.5,4.5; A5 7.5,3.5; A6 7.5,2.5; A7 7.5,1.5; A8 7.5,0.5; A9 7.5,-0.5; A10 7.5,-1.5; A11 7.5,-2.5; A12 7.5,-3.5; A13 7.5,-4.5; A14 7.5,-5.5; A15 7.5,-6.5; A16 7.5,-7.5; B1 6.5,7.5; B2 6.5,6.5; B3 6.5,5.5; B4 6.5,4.5; B5 6.5,3.5; B6 6.5,2.5; B7 6.5,1.5; B8 6.5,0.5; B9 6.5,-0.5; B10 6.5,-1.5; B11 6.5,-2.5; B12 6.5,-3.5; B13 6.5,-4.5; B14 6.5,-5.5; B15 6.5,-6.5; B16 6.5,-7.5; C1 5.5,7.5; C2 5.5,6.5; C3 5.5,5.5; C4 5.5,4.5; C5 5.5,3.5; C6 5.5,2.5; C7 5.5,1.5; C8 5.5,0.5; C9 5.5,-0.5; C10 5.5,-1.5; C11 5.5,-2.5; C12 5.5,-3.5; C13 5.5,-4.5; C14 5.5,-5.5; C15 5.5,-6.5; C16 5.5,-7.5; D1 4.5,7.5; D2 4.5,6.5; D3 4.5,5.5; D4 4.5,4.5; D5 4.5,3.5; D6 4.5,2.5; D7 4.5,1.5; D8 4.5,0.5; D9 4.5,-0.5; D10 4.5,-1.5; D11 4.5,-2.5; D12 4.5,-3.5; D13 4.5,-4.5; D14 4.5,-5.5; D15 4.5,-6.5; D16 4.5,-7.5; E1 3.5,7.5; E2 3.5,6.5; E3 3.5,5.5; E4 3.5,4.5; E5 3.5,3.5; E6 3.5,2.5; E7 3.5,1.5; E8 3.5,0.5; E9 3.5,-0.5; E10 3.5,-1.5; E11 3.5,-2.5; E12 3.5,-3.5; E13 3.5,-4.5; E14 3.5,-5.5; E15 3.5,-6.5; E16 3.5,-7.5; F1 2.5,7.5; F2 2.5,6.5; F3 2.5,5.5; F4 2.5,4.5; F5 2.5,3.5; F6 2.5,2.5; F7 2.5,1.5; F8 2.5,0.5; F9 2.5,-0.5; F10 2.5,-1.5; F11 2.5,-2.5; F12 2.5,-3.5; F13 2.5,-4.5; F14 2.5,-5.5; F15 2.5,-6.5; F16 2.5,-7.5; G1 1.5,7.5; G2 1.5,6.5; G3 1.5,5.5; G4 1.5,4.5; G5 1.5,3.5; G6 1.5,2.5; G7 1.5,1.5; G8 1.5,0.5; G9 1.5,-0.5; G10 1.5,-1.5; G11 1.5,-2.5; G12 1.5,-3.5; G13 1.5,-4.5; G14 1.5,-5.5; G15 1.5,-6.5; G16 1.5,-7.5; H1 0.5,7.5; H2 0.5,6.5; H3 0.5,5.5; H4 0.5,4.5; H5 0.5,3.5; H6 0.5,2.5; H7 0.5,1.5; H8 0.5,0.5; H9 0.5,-0.5; H10 0.5,-1.5; H11 0.5,-2.5; H12 0.5,-3.5; H13 0.5,-4.5; H14 0.5,-5.5; H15 0.5,-6.5; H16 0.5,-7.5; J1 -0.5,7.5; J2 -0.5,6.5; J3 -0.5,5.5; J4 -0.5,4.5; J5 -0.5,3.5; J6 -0.5,2.5; J7 -0.5,1.5; J8 -0.5,0.5; J9 -0.5,-0.5; J10 -0.5,-1.5; J11 -0.5,-2.5; J12 -0.5,-3.5; J13 -0.5,-4.5; J14 -0.5,-5.5; J15 -0.5,-6.5; J16 -0.5,-7.5; K1 -1.5,7.5; K2 -1.5,6.5; K3 -1.5,5.5; K4 -1.5,4.5; K5 -1.5,3.5; K6 -1.5,2.5; K7 -1.5,1.5; K8 -1.5,0.5; K9 -1.5,-0.5; K10 -1.5,-1.5; K11 -1.5,-2.5; K12 -1.5,-3.5; K13 -1.5,-4.5; K14 -1.5,-5.5; K15 -1.5,-6.5; K16 -1.5,-7.5; L1 -2.5,7.5; L2 -2.5,6.5; L3 -2.5,5.5; L4 -2.5,4.5; L5 -2.5,3.5; L6 -2.5,2.5; L7 -2.5,1.5; L8 -2.5,0.5; L9 -2.5,-0.5; L10 -2.5,-1.5; L11 -2.5,-2.5; L12 -2.5,-3.5; L13 -2.5,-4.5; L14 -2.5,-5.5; L15 -2.5,-6.5; L16 -2.5,-7.5; M1 -3.5,7.5; M2 -3.5,6.5; M3 -3.5,5.5; M4 -3.5,4.5; M5 -3.5,3.5; M6 -3.5,2.5; M7 -3.5,1.5; M8 -3.5,0.5; M9 -3.5,-0.5; M10 -3.5,-1.5; M11 -3.5,-2.5; M12 -3.5,-3.5; M13 -3.5,-4.5; M14 -3.5,-5.5; M15 -3.5,-6.5; M16 -3.5,-7.5; N1 -4.5,7.5; N2 -4.5,6.5; N3 -4.5,5.5; N4 -4.5,4.5; N5 -4.5,3.5; N6 -4.5,2.5; N7 -4.5,1.5; N8 -4.5,0.5; N9 -4.5,-0.5; N10 -4.5,-1.5; N11 -4.5,-2.5; N12 -4.5,-3.5; N13 -4.5,-4.5; N14 -4.5,-5.5; N15 -4.5,-6.5; N16 -4.5,-7.5; P1 -5.5,7.5; P2 -5.5,6.5; P3 -5.5,5.5; P4 -5.5,4.5; P5 -5.5,3.5; P6 -5.5,2.5; P7 -5.5,1.5; P8 -5.5,0.5; P9 -5.5,-0.5; P10 -5.5,-1.5; P11 -5.5,-2.5; P12 -5.5,-3.5; P13 -5.5,-4.5; P14 -5.5,-5.5; P15 -5.5,-6.5; P16 -5.5,-7.5; R1 -6.5,7.5; R2 -6.5,6.5; R3 -6.5,5.5; R4 -6.5,4.5; R5 -6.5,3.5; R6 -6.5,2.5; R7 -6.5,1.5; R8 -6.5,0.5; R9 -6.5,-0.5; R10 -6.5,-1.5; R11 -6.5,-2.5; R12 -6.5,-3.5; R13 -6.5,-4.5; R14 -6.5,-5.5; R15 -6.5,-6.5; R16 -6.5,-7.5; T1 -7.5,7.5; T2 -7.5,6.5; T3 -7.5,5.5; T4 -7.5,4.5; T5 -7.5,3.5; T6 -7.5,2.5; T7 -7.5,1.5; T8 -7.5,0.5; T9 -7.5,-0.5; T10 -7.5,-1.5; T11 -7.5,-2.5; T12 -7.5,-3.5; T13 -7.5,-4.5; T14 -7.5,-5.5; T15 -7.5,-6.5; T16 -7.5,-7.5 | hole 1.47: 13.6,-8.45; -13.6,8.45 | hole 2.26: -19.6,10.75; -19.6,-10.75; 19.6,-10.75; 19.6,10.75
SOD-123 = smd 1.4 x 1.4: A 1.85,0; C -1.85,0
SOD-323 = smd 1.35 x 0.8: A 1.27,0; C -1.27,0
SOD-523 = smd 0.8 x 0.6: A 0,-0.75; K 0,0.75
SOIC-4 = smd 1.2 x 1.2: + 1.3,3.05; - -1.3,3.05; ~1 -1.3,-3.05; ~2 1.3,-3.05
SOIC8_150MIL = smd 0.6 x 2.2: 1 -1.905,-2.6; 2 -0.635,-2.6; 3 0.635,-2.6; 4 1.905,-2.6; 5 1.905,2.6; 6 0.635,2.6; 7 -0.635,2.6; 8 -1.905,2.6
SOIC8_208MIL = smd 0.6 x 2.2: 1 -1.905,-3.315; 2 -0.635,-3.315; 3 0.635,-3.315; 4 1.905,-3.315; 5 1.905,3.315; 6 0.635,3.315; 7 -0.635,3.315; 8 -1.905,3.315
SOIC14 = smd 0.6 x 2.2: 1 -3.81,-2.6; 2 -2.54,-2.6; 3 -1.27,-2.6; 4 0,-2.6; 5 1.27,-2.6; 6 2.54,-2.6; 7 3.81,-2.6; 8 3.81,2.6; 9 2.54,2.6; 10 1.27,2.6; 11 0,2.6; 12 -1.27,2.6; 13 -2.54,2.6; 14 -3.81,2.6
SOIC16 = smd 0.6 x 2.2: 1 -4.445,-2.6; 2 -3.175,-2.6; 3 -1.905,-2.6; 4 -0.635,-2.6; 5 0.635,-2.6; 6 1.905,-2.6; 7 3.175,-2.6; 8 4.445,-2.6; 9 4.445,2.6; 10 3.175,2.6; 11 1.905,2.6; 12 0.635,2.6; 13 -0.635,2.6; 14 -1.905,2.6; 15 -3.175,2.6; 16 -4.445,2.6
SOIC20WIDE = smd 0.66 x 2.032: 1 -5.715,-5.029; 2 -4.445,-5.029; 3 -3.175,-5.029; 4 -1.905,-5.029; 5 -0.635,-5.029; 6 0.635,-5.029; 7 1.905,-5.029; 8 3.175,-5.029; 9 4.445,-5.029; 10 5.715,-5.029; 11 5.715,5.029; 12 4.445,5.029; 13 3.175,5.029; 14 1.905,5.029; 15 0.635,5.029; 16 -0.635,5.029; 17 -1.905,5.029; 18 -3.175,5.029; 19 -4.445,5.029; 20 -5.715,5.029
SOIC24WIDE = smd 0.66 x 2.032: 1 -6.985,-5.029; 2 -5.715,-5.029; 3 -4.445,-5.029; 4 -3.175,-5.029; 5 -1.905,-5.029; 6 -0.635,-5.029; 7 0.635,-5.029; 8 1.905,-5.029; 9 3.175,-5.029; 10 4.445,-5.029; 11 5.715,-5.029; 12 6.985,-5.029; 13 6.985,5.029; 14 5.715,5.029; 15 4.445,5.029; 16 3.175,5.029; 17 1.905,5.029; 18 0.635,5.029; 19 -0.635,5.029; 20 -1.905,5.029; 21 -3.175,5.029; 22 -4.445,5.029; 23 -5.715,5.029; 24 -6.985,5.029
SOLDERJUMPER_2WAY_OPEN_0603 = smd 1.1 x 1: 1 -1.7,0; 2 0,0; 3 1.7,0
SOLDERJUMPER_2WAY_OPEN_0805 = smd 1.3 x 1.5: 1 -1.9,0; 2 0,0; 3 1.9,0
SOLDERJUMPER_2WAY_OPEN_NOPASTE = smd 1.168 x 1.6: 1 -1.397,0; 2 1.397,0; 3 0,0
SOLDERJUMPER_ARROW_NOPASTE = smd 0.762 x 1.524: 1 -1.016,0; 2 1.016,0
SOLDERJUMPER_CLOSEDPERM = smd 1.168 x 1.6: 1 -0.762,0; 2 0.762,0 | smd 0.635 x 1.6: WIRE 0,0
SOLDERJUMPER_CLOSEDWIRE = smd 1.168 x 1.6: 1 -0.762,0; 2 0.762,0 | smd 0.635 x 0.203: WIRE 0,0
SOLDERJUMPER_REFLOW = smd 1.168 x 1.6: 1 -0.762,0; 2 0.762,0
SOLDERJUMPER_REFLOW_NOPASTE = smd 1.168 x 1.6: 1 -0.762,0; 2 0.762,0
SOLDERJUMPER_WAVE = smd 1.27 x 2.54: 1 -1.27,0; 2 1.27,0
SOP8-1351 = smd 2.54 x 1.524: 1 -8.382,3.81; 2 -8.382,1.27; 3 -8.382,-1.27; 4 -8.382,-3.81; 5 8.382,-3.81; 6 8.382,-1.27; 7 8.382,1.27; 8 8.382,3.81
SOP8-1369 = smd 2.54 x 1.524: 1 -8.382,3.81; 2 -8.382,1.27; 3 -8.382,-1.27; 4 -8.382,-3.81; 5 8.382,-3.81; 6 8.382,-1.27; 7 8.382,1.27; 8 8.382,3.81
SOP20_300MIL = smd 0.635 x 2.286: P$1 -5.715,-5.08; P$2 -4.445,-5.08; P$3 -3.175,-5.08; P$4 -1.905,-5.08; P$5 -0.635,-5.08; P$6 0.635,-5.08; P$7 1.905,-5.08; P$8 3.175,-5.08; P$9 4.445,-5.08; P$10 5.715,-5.08; P$11 5.715,5.08; P$12 4.445,5.08; P$13 3.175,5.08; P$14 1.905,5.08; P$15 0.635,5.08; P$16 -0.635,5.08; P$17 -1.905,5.08; P$18 -3.175,5.08; P$19 -4.445,5.08; P$20 -5.715,5.08
SOP24_300MIL = smd 0.635 x 2.286: P$1 -6.985,-5.08; P$2 -5.715,-5.08; P$3 -4.445,-5.08; P$4 -3.175,-5.08; P$5 -1.905,-5.08; P$6 -0.635,-5.08; P$7 0.635,-5.08; P$8 1.905,-5.08; P$9 3.175,-5.08; P$10 4.445,-5.08; P$11 5.715,-5.08; P$12 6.985,-5.08; P$13 6.985,5.08; P$14 5.715,5.08; P$15 4.445,5.08; P$16 3.175,5.08; P$17 1.905,5.08; P$18 0.635,5.08; P$19 -0.635,5.08; P$20 -1.905,5.08; P$21 -3.175,5.08; P$22 -4.445,5.08; P$23 -5.715,5.08; P$24 -6.985,5.08
SOP28_300MIL = smd 0.635 x 2.286: P$1 -8.255,-5.08; P$2 -6.985,-5.08; P$3 -5.715,-5.08; P$4 -4.445,-5.08; P$5 -3.175,-5.08; P$6 -1.905,-5.08; P$7 -0.635,-5.08; P$8 0.635,-5.08; P$9 1.905,-5.08; P$10 3.175,-5.08; P$11 4.445,-5.08; P$12 5.715,-5.08; P$13 6.985,-5.08; P$14 8.255,-5.08; P$15 8.255,5.08; P$16 6.985,5.08; P$17 5.715,5.08; P$18 4.445,5.08; P$19 3.175,5.08; P$20 1.905,5.08; P$21 0.635,5.08; P$22 -0.635,5.08; P$23 -1.905,5.08; P$24 -3.175,5.08; P$25 -4.445,5.08; P$26 -5.715,5.08; P$27 -6.985,5.08; P$28 -8.255,5.08
SOT23-5 = smd 0.55 x 1.2: 1 -0.95,-1.3; 2 0,-1.3; 3 0.95,-1.3; 4 0.95,1.3; 5 -0.95,1.3
SOT23-6 = smd 0.55 x 1.2: 1 -0.95,-1.3; 2 0,-1.3; 3 0.95,-1.3; 4 0.95,1.3; 5 0,1.3; 6 -0.95,1.3
SOT23-8 = smd 0.4 x 1.2: 1 -0.975,-1.3; 2 -0.325,-1.3; 3 0.325,-1.3; 4 0.975,-1.3; 5 0.975,1.3; 6 0.325,1.3; 7 -0.325,1.3; 8 -0.975,1.3
SOT23-R = smd 0.635 x 1.016: 1 -0.95,-1; 2 0.95,-1; 3 0,1
SOT23-W = smd 1.2 x 1.4: 1 -1.1,-1.3; 2 1.1,-1.3 | smd 2.8 x 1.4: 3 0,1.3
SOT23-WIDE = smd 1 x 1.27: 1 -0.95,-1; 2 0.95,-1; 3 0,1
SOT223-R = smd 1.3 x 1.3: 1 -2.3,-3.05; 2 0,-3.05; 3 2.3,-3.05 | smd 3.6 x 1.3: 4 0,3.05
SOT223-W = smd 1.9 x 1.9: 1 -2.7,-3.1; 3 2.7,-3.1 | smd 1.1 x 1.9: 2 0,-3.1 | smd 6.7 x 1.9: 4 0,3.1
SOT323-R = smd 0.6 x 0.55: 1 -0.65,-0.925; 2 0.65,-0.925; 3 0,0.925
SOT323-W = smd 0.9 x 1.45: 1 -0.9,-1.275; 2 0.9,-1.275 | smd 2.1 x 1.45: 3 0,1.275
SOT363 = smd 0.5 x 0.5: 1 -0.75,-0.9; 3 0.75,-0.9; 4 0.75,0.9; 6 -0.75,0.9 | smd 0.4 x 0.5: 2 0,-0.9; 5 0,0.9
SOT833-1 = smd 0.4 x 0.25: 1 0.275,-0.75 | smd 0.35 x 0.25: 2 0.3,-0.25; 3 0.3,0.25; 4 0.3,0.75; 5 -0.3,0.75; 6 -0.3,0.25; 7 -0.3,-0.25; 8 -0.3,-0.75
SOT886 = smd 0.325 x 0.27: 1 -0.338,0.5; 2 -0.338,0; 3 -0.338,-0.5; 4 0.338,-0.5; 5 0.338,0; 6 0.338,0.5
SPDT_SMT_SSSS811101 = smd 0.7 x 1.5: A -2.25,1.75; B 0.75,1.75; C 2.25,1.75 | smd 1 x 0.8: SUP1 -3.65,1.1; SUP2 -3.65,-1.1; SUP3 3.65,1.1; SUP4 3.65,-1.1 | hole 0.9: -1.5,0; 1.5,0
SPST_SMT_19192 = smd 0.7 x 1.5: A -2.25,1.75; B 0.75,1.75; C 2.25,1.75 | smd 1 x 0.8: GND1 -3.65,1; GND2 -3.65,-1; GND3 3.65,1; GND4 3.65,-1 | hole 0.9: -1.5,0; 1.5,0
SSOP24 = smd 0.4 x 1.2: 1 -3.575,-3.42; 2 -2.925,-3.42; 3 -2.275,-3.42; 4 -1.625,-3.42; 5 -0.975,-3.42; 6 -0.325,-3.42; 7 0.325,-3.42; 8 0.975,-3.42; 9 1.625,-3.42; 10 2.275,-3.42; 11 2.925,-3.42; 12 3.575,-3.42; 13 3.575,3.42; 14 2.925,3.42; 15 2.275,3.42; 16 1.625,3.42; 17 0.975,3.42; 18 0.325,3.42; 19 -0.325,3.42; 20 -0.975,3.42; 21 -1.625,3.42; 22 -2.275,3.42; 23 -2.925,3.42; 24 -3.575,3.42
SSOP28DB = smd 0.348 x 1.397: 1 -4.225,-3.656; 2 -3.575,-3.656; 3 -2.925,-3.656; 4 -2.275,-3.656; 5 -1.625,-3.656; 6 -0.975,-3.656; 7 -0.325,-3.656; 8 0.325,-3.656; 9 0.975,-3.656; 10 1.625,-3.656; 11 2.275,-3.656; 12 2.925,-3.656; 13 3.575,-3.656; 14 4.225,-3.656; 15 4.225,3.656; 16 3.575,3.656; 17 2.925,3.656; 18 2.275,3.656; 19 1.625,3.656; 20 0.975,3.656; 21 0.325,3.656; 22 -0.325,3.656; 23 -0.975,3.656; 24 -1.625,3.656; 25 -2.275,3.656; 26 -2.925,3.656; 27 -3.575,3.656; 28 -4.225,3.656
STANDARDCONNECTOR = drill 1 square: 1 -11.43,-1.27 | drill 1: 2 -11.43,1.27; 3 -8.89,-1.27; 4 -8.89,1.27; 5 -6.35,-1.27; 6 -6.35,1.27; 7 -3.81,-1.27; 8 -3.81,1.27; 9 -1.27,-1.27; 10 -1.27,1.27; 11 1.27,-1.27; 12 1.27,1.27; 13 3.81,-1.27; 14 3.81,1.27; 15 6.35,-1.27; 16 6.35,1.27; 17 8.89,-1.27; 18 8.89,1.27; 19 11.43,-1.27; 20 11.43,1.27
STX3100 = drill 1.5 pad 2.54: 1 2.7,-0.1 | drill 1.5: 2 7.7,5; 3 7.7,2.3; 4 7.7,-2.5; 5 7.7,-5.2 | hole 1.5: 2.7,4.9; 2.7,-5.1; 7.7,-0.1
SWITCH_4WAY_TPA511GLFS = smd 1 x 1.4: COMMON1 -5.825,-4.3; COMMON2 -5.825,-2.6; DOWN/4 3.25,-4.3; LEFT/7 -5.825,1.7; RIGHT/6 -5.825,0; SELECT/5 3.25,1.7; UP/3 3.25,-2.6 | hole 0.6: -2.7,0.5 | hole 0.9: 1.5,-2.7
TCS3414_CS6 = smd 0.3 x 0.3: A1 -0.61,0.475; A2 0,0.475; A3 0.61,0.475; B1 -0.61,-0.475; B2 0,-0.475; B3 0.61,-0.475
TDFN14_3X3MM = smd 0.7 x 0.2: P$1 -1.475,1.2; P$2 -1.475,0.8; P$3 -1.475,0.4; P$4 -1.475,0; P$5 -1.475,-0.4; P$6 -1.475,-0.8; P$7 -1.475,-1.2; P$8 1.475,-1.2; P$9 1.475,-0.8; P$10 1.475,-0.4; P$11 1.475,0; P$12 1.475,0.4; P$13 1.475,0.8; P$14 1.475,1.2 | smd 1.27 x 2.35: P$THERMAL 0,0
TEA5767MODULE = smd 1.016 x 2.54: 1 -4.064,-5.588; 2 -2.032,-5.588; 3 0,-5.588; 4 2.032,-5.588; 5 4.064,-5.588; 6 4.064,5.588; 7 2.032,5.588; 8 0,5.588; 9 -2.032,5.588; 10 -4.064,5.588
TERMBLOCK_1X2-3.5MM = drill 1 pad 2.184: 1 1.8,0; 2 -1.7,0
TERMBLOCK_1X3-3.5MM = drill 1 pad 2.184: 1 3.55,0; 2 0.05,0; 3 -3.45,0
TESTPOINT_PAD_2MM = smd 2 x 2: P$1 0,0
TESTPOINT_ROUND_0.5MM = smd 0.5 x 0.5: P$1 0,0
TESTPOINT_ROUND_1MM = smd 1 x 1: P$1 0,0
TESTPOINT_ROUND_2MM = smd 2 x 2: P$1 0,0
TESTPOINT_SMT = smd 4.7 x 3.4: P$1 0,0
TFBGA100_0.8 = smd 0.34 x 0.34: A1 -3.6,3.6; A2 -2.8,3.6; A3 -2,3.6; A4 -1.2,3.6; A5 -0.4,3.6; A6 0.4,3.6; A7 1.2,3.6; A8 2,3.6; A9 2.8,3.6; A10 3.6,3.6; B1 -3.6,2.8; B2 -2.8,2.8; B3 -2,2.8; B4 -1.2,2.8; B5 -0.4,2.8; B6 0.4,2.8; B7 1.2,2.8; B8 2,2.8; B9 2.8,2.8; B10 3.6,2.8; C1 -3.6,2; C2 -2.8,2; C3 -2,2; C4 -1.2,2; C5 -0.4,2; C6 0.4,2; C7 1.2,2; C8 2,2; C9 2.8,2; C10 3.6,2; D1 -3.6,1.2; D2 -2.8,1.2; D3 -2,1.2; D4 -1.2,1.2; D5 -0.4,1.2; D6 0.4,1.2; D7 1.2,1.2; D8 2,1.2; D9 2.8,1.2; D10 3.6,1.2; E1 -3.6,0.4; E2 -2.8,0.4; E3 -2,0.4; E4 -1.2,0.4; E5 -0.4,0.4; E6 0.4,0.4; E7 1.2,0.4; E8 2,0.4; E9 2.8,0.4; E10 3.6,0.4; F1 -3.6,-0.4; F2 -2.8,-0.4; F3 -2,-0.4; F4 -1.2,-0.4; F5 -0.4,-0.4; F6 0.4,-0.4; F7 1.2,-0.4; F8 2,-0.4; F9 2.8,-0.4; F10 3.6,-0.4; G1 -3.6,-1.2; G2 -2.8,-1.2; G3 -2,-1.2; G4 -1.2,-1.2; G5 -0.4,-1.2; G6 0.4,-1.2; G7 1.2,-1.2; G8 2,-1.2; G9 2.8,-1.2; G10 3.6,-1.2; H1 -3.6,-2; H2 -2.8,-2; H3 -2,-2; H4 -1.2,-2; H5 -0.4,-2; H6 0.4,-2; H7 1.2,-2; H8 2,-2; H9 2.8,-2; H10 3.6,-2; J1 -3.6,-2.8; J2 -2.8,-2.8; J3 -2,-2.8; J4 -1.2,-2.8; J5 -0.4,-2.8; J6 0.4,-2.8; J7 1.2,-2.8; J8 2,-2.8; J9 2.8,-2.8; J10 3.6,-2.8; K1 -3.6,-3.6; K2 -2.8,-3.6; K3 -2,-3.6; K4 -1.2,-3.6; K5 -0.4,-3.6; K6 0.4,-3.6; K7 1.2,-3.6; K8 2,-3.6; K9 2.8,-3.6; K10 3.6,-3.6
TFBGA180_0.8 = smd 0.34 x 0.34: A1 -5.2,5.2; A2 -4.4,5.2; A3 -3.6,5.2; A4 -2.8,5.2; A5 -2,5.2; A6 -1.2,5.2; A7 -0.4,5.2; A8 0.4,5.2; A9 1.2,5.2; A10 2,5.2; A11 2.8,5.2; A12 3.6,5.2; A13 4.4,5.2; A14 5.2,5.2; B1 -5.2,4.4; B2 -4.4,4.4; B3 -3.6,4.4; B4 -2.8,4.4; B5 -2,4.4; B6 -1.2,4.4; B7 -0.4,4.4; B8 0.4,4.4; B9 1.2,4.4; B10 2,4.4; B11 2.8,4.4; B12 3.6,4.4; B13 4.4,4.4; B14 5.2,4.4; C1 -5.2,3.6; C2 -4.4,3.6; C3 -3.6,3.6; C4 -2.8,3.6; C5 -2,3.6; C6 -1.2,3.6; C7 -0.4,3.6; C8 0.4,3.6; C9 1.2,3.6; C10 2,3.6; C11 2.8,3.6; C12 3.6,3.6; C13 4.4,3.6; C14 5.2,3.6; D1 -5.2,2.8; D2 -4.4,2.8; D3 -3.6,2.8; D4 -2.8,2.8; D5 -2,2.8; D6 -1.2,2.8; D7 -0.4,2.8; D8 0.4,2.8; D9 1.2,2.8; D10 2,2.8; D11 2.8,2.8; D12 3.6,2.8; D13 4.4,2.8; D14 5.2,2.8; E1 -5.2,2; E2 -4.4,2; E3 -3.6,2; E4 -2.8,2; E5 -2,2; E6 -1.2,2; E7 -0.4,2; E8 0.4,2; E9 1.2,2; E10 2,2; E11 2.8,2; E12 3.6,2; E13 4.4,2; E14 5.2,2; F1 -5.2,1.2; F2 -4.4,1.2; F3 -3.6,1.2; F4 -2.8,1.2; F5 -2,1.2; F10 2,1.2; F11 2.8,1.2; F12 3.6,1.2; F13 4.4,1.2; F14 5.2,1.2; G1 -5.2,0.4; G2 -4.4,0.4; G3 -3.6,0.4; G4 -2.8,0.4; G5 -2,0.4; G10 2,0.4; G11 2.8,0.4; G12 3.6,0.4; G13 4.4,0.4; G14 5.2,0.4; H1 -5.2,-0.4; H2 -4.4,-0.4; H3 -3.6,-0.4; H4 -2.8,-0.4; H5 -2,-0.4; H10 2,-0.4; H11 2.8,-0.4; H12 3.6,-0.4; H13 4.4,-0.4; H14 5.2,-0.4; J1 -5.2,-1.2; J2 -4.4,-1.2; J3 -3.6,-1.2; J4 -2.8,-1.2; J5 -2,-1.2; J10 2,-1.2; J11 2.8,-1.2; J12 3.6,-1.2; J13 4.4,-1.2; J14 5.2,-1.2; K1 -5.2,-2; K2 -4.4,-2; K3 -3.6,-2; K4 -2.8,-2; K5 -2,-2; K6 -1.2,-2; K7 -0.4,-2; K8 0.4,-2; K9 1.2,-2; K10 2,-2; K11 2.8,-2; K12 3.6,-2; K13 4.4,-2; K14 5.2,-2; L1 -5.2,-2.8; L2 -4.4,-2.8; L3 -3.6,-2.8; L4 -2.8,-2.8; L5 -2,-2.8; L6 -1.2,-2.8; L7 -0.4,-2.8; L8 0.4,-2.8; L9 1.2,-2.8; L10 2,-2.8; L11 2.8,-2.8; L12 3.6,-2.8; L13 4.4,-2.8; L14 5.2,-2.8; M1 -5.2,-3.6; M2 -4.4,-3.6; M3 -3.6,-3.6; M4 -2.8,-3.6; M5 -2,-3.6; M6 -1.2,-3.6; M7 -0.4,-3.6; M8 0.4,-3.6; M9 1.2,-3.6; M10 2,-3.6; M11 2.8,-3.6; M12 3.6,-3.6; M13 4.4,-3.6; M14 5.2,-3.6; N1 -5.2,-4.4; N2 -4.4,-4.4; N3 -3.6,-4.4; N4 -2.8,-4.4; N5 -2,-4.4; N6 -1.2,-4.4; N7 -0.4,-4.4; N8 0.4,-4.4; N9 1.2,-4.4; N10 2,-4.4; N11 2.8,-4.4; N12 3.6,-4.4; N13 4.4,-4.4; N14 5.2,-4.4; P1 -5.2,-5.2; P2 -4.4,-5.2; P3 -3.6,-5.2; P4 -2.8,-5.2; P5 -2,-5.2; P6 -1.2,-5.2; P7 -0.4,-5.2; P8 0.4,-5.2; P9 1.2,-5.2; P10 2,-5.2; P11 2.8,-5.2; P12 3.6,-5.2; P13 4.4,-5.2; P14 5.2,-5.2
TFBGA208_0.8 = smd 0.34 x 0.34: A1 -6.4,6.4; A2 -5.6,6.4; A3 -4.8,6.4; A4 -4,6.4; A5 -3.2,6.4; A6 -2.4,6.4; A7 -1.6,6.4; A8 -0.8,6.4; A9 0,6.4; A10 0.8,6.4; A11 1.6,6.4; A12 2.4,6.4; A13 3.2,6.4; A14 4,6.4; A15 4.8,6.4; A16 5.6,6.4; A17 6.4,6.4; B1 -6.4,5.6; B2 -5.6,5.6; B3 -4.8,5.6; B4 -4,5.6; B5 -3.2,5.6; B6 -2.4,5.6; B7 -1.6,5.6; B8 -0.8,5.6; B9 0,5.6; B10 0.8,5.6; B11 1.6,5.6; B12 2.4,5.6; B13 3.2,5.6; B14 4,5.6; B15 4.8,5.6; B16 5.6,5.6; B17 6.4,5.6; C1 -6.4,4.8; C2 -5.6,4.8; C3 -4.8,4.8; C4 -4,4.8; C5 -3.2,4.8; C6 -2.4,4.8; C7 -1.6,4.8; C8 -0.8,4.8; C9 0,4.8; C10 0.8,4.8; C11 1.6,4.8; C12 2.4,4.8; C13 3.2,4.8; C14 4,4.8; C15 4.8,4.8; C16 5.6,4.8; C17 6.4,4.8; D1 -6.4,4; D2 -5.6,4; D3 -4.8,4; D4 -4,4; D5 -3.2,4; D6 -2.4,4; D7 -1.6,4; D8 -0.8,4; D9 0,4; D10 0.8,4; D11 1.6,4; D12 2.4,4; D13 3.2,4; D14 4,4; D15 4.8,4; D16 5.6,4; D17 6.4,4; E1 -6.4,3.2; E2 -5.6,3.2; E3 -4.8,3.2; E4 -4,3.2; E14 4,3.2; E15 4.8,3.2; E16 5.6,3.2; E17 6.4,3.2; F1 -6.4,2.4; F2 -5.6,2.4; F3 -4.8,2.4; F4 -4,2.4; F14 4,2.4; F15 4.8,2.4; F16 5.6,2.4; F17 6.4,2.4; G1 -6.4,1.6; G2 -5.6,1.6; G3 -4.8,1.6; G4 -4,1.6; G14 4,1.6; G15 4.8,1.6; G16 5.6,1.6; G17 6.4,1.6; H1 -6.4,0.8; H2 -5.6,0.8; H3 -4.8,0.8; H4 -4,0.8; H14 4,0.8; H15 4.8,0.8; H16 5.6,0.8; H17 6.4,0.8; J1 -6.4,0; J2 -5.6,0; J3 -4.8,0; J4 -4,0; J14 4,0; J15 4.8,0; J16 5.6,0; J17 6.4,0; K1 -6.4,-0.8; K2 -5.6,-0.8; K3 -4.8,-0.8; K4 -4,-0.8; K14 4,-0.8; K15 4.8,-0.8; K16 5.6,-0.8; K17 6.4,-0.8; L1 -6.4,-1.6; L2 -5.6,-1.6; L3 -4.8,-1.6; L4 -4,-1.6; L14 4,-1.6; L15 4.8,-1.6; L16 5.6,-1.6; L17 6.4,-1.6; M1 -6.4,-2.4; M2 -5.6,-2.4; M3 -4.8,-2.4; M4 -4,-2.4; M14 4,-2.4; M15 4.8,-2.4; M16 5.6,-2.4; M17 6.4,-2.4; N1 -6.4,-3.2; N2 -5.6,-3.2; N3 -4.8,-3.2; N4 -4,-3.2; N14 4,-3.2; N15 4.8,-3.2; N16 5.6,-3.2; N17 6.4,-3.2; P1 -6.4,-4; P2 -5.6,-4; P3 -4.8,-4; P4 -4,-4; P5 -3.2,-4; P6 -2.4,-4; P7 -1.6,-4; P8 -0.8,-4; P9 0,-4; P10 0.8,-4; P11 1.6,-4; P12 2.4,-4; P13 3.2,-4; P14 4,-4; P15 4.8,-4; P16 5.6,-4; P17 6.4,-4; R1 -6.4,-4.8; R2 -5.6,-4.8; R3 -4.8,-4.8; R4 -4,-4.8; R5 -3.2,-4.8; R6 -2.4,-4.8; R7 -1.6,-4.8; R8 -0.8,-4.8; R9 0,-4.8; R10 0.8,-4.8; R11 1.6,-4.8; R12 2.4,-4.8; R13 3.2,-4.8; R14 4,-4.8; R15 4.8,-4.8; R16 5.6,-4.8; R17 6.4,-4.8; T1 -6.4,-5.6; T2 -5.6,-5.6; T3 -4.8,-5.6; T4 -4,-5.6; T5 -3.2,-5.6; T6 -2.4,-5.6; T7 -1.6,-5.6; T8 -0.8,-5.6; T9 0,-5.6; T10 0.8,-5.6; T11 1.6,-5.6; T12 2.4,-5.6; T13 3.2,-5.6; T14 4,-5.6; T15 4.8,-5.6; T16 5.6,-5.6; T17 6.4,-5.6; U1 -6.4,-6.4; U2 -5.6,-6.4; U3 -4.8,-6.4; U4 -4,-6.4; U5 -3.2,-6.4; U6 -2.4,-6.4; U7 -1.6,-6.4; U8 -0.8,-6.4; U9 0,-6.4; U10 0.8,-6.4; U11 1.6,-6.4; U12 2.4,-6.4; U13 3.2,-6.4; U14 4,-6.4; U15 4.8,-6.4; U16 5.6,-6.4; U17 6.4,-6.4
TFBGA208_0.65 = smd 0.25 x 0.25: 15 3.9,-1.95; A1 -5.2,5.2; A2 -4.55,5.2; A3 -3.9,5.2; A4 -3.25,5.2; A5 -2.6,5.2; A6 -1.95,5.2; A7 -1.3,5.2; A8 -0.65,5.2; A9 0,5.2; A10 0.65,5.2; A11 1.3,5.2; A12 1.95,5.2; A13 2.6,5.2; A14 3.25,5.2; A15 3.9,5.2; A16 4.55,5.2; A17 5.2,5.2; B1 -5.2,4.55; B2 -4.55,4.55; B3 -3.9,4.55; B4 -3.25,4.55; B5 -2.6,4.55; B6 -1.95,4.55; B7 -1.3,4.55; B8 -0.65,4.55; B9 0,4.55; B10 0.65,4.55; B11 1.3,4.55; B12 1.95,4.55; B13 2.6,4.55; B14 3.25,4.55; B15 3.9,4.55; B16 4.55,4.55; B17 5.2,4.55; C1 -5.2,3.9; C2 -4.55,3.9; C3 -3.9,3.9; C4 -3.25,3.9; C5 -2.6,3.9; C6 -1.95,3.9; C7 -1.3,3.9; C8 -0.65,3.9; C9 0,3.9; C10 0.65,3.9; C11 1.3,3.9; C12 1.95,3.9; C13 2.6,3.9; C14 3.25,3.9; C15 3.9,3.9; C16 4.55,3.9; C17 5.2,3.9; D1 -5.2,3.25; D2 -4.55,3.25; D3 -3.9,3.25; D4 -3.25,3.25; D5 -2.6,3.25; D6 -1.95,3.25; D7 -1.3,3.25; D8 -0.65,3.25; D9 0,3.25; D10 0.65,3.25; D11 1.3,3.25; D12 1.95,3.25; D13 2.6,3.25; D14 3.25,3.25; D15 3.9,3.25; D16 4.55,3.25; D17 5.2,3.25; E1 -5.2,2.6; E2 -4.55,2.6; E3 -3.9,2.6; E4 -3.25,2.6; E14 3.25,2.6; E15 3.9,2.6; E16 4.55,2.6; E17 5.2,2.6; F1 -5.2,1.95; F2 -4.55,1.95; F3 -3.9,1.95; F4 -3.25,1.95; F14 3.25,1.95; F15 3.9,1.95; F16 4.55,1.95; F17 5.2,1.95; G1 -5.2,1.3; G2 -4.55,1.3; G3 -3.9,1.3; G4 -3.25,1.3; G14 3.25,1.3; G15 3.9,1.3; G16 4.55,1.3; G17 5.2,1.3; H1 -5.2,0.65; H2 -4.55,0.65; H3 -3.9,0.65; H4 -3.25,0.65; H14 3.25,0.65; H15 3.9,0.65; H16 4.55,0.65; H17 5.2,0.65; J1 -5.2,0; J2 -4.55,0; J3 -3.9,0; J4 -3.25,0; J14 3.25,0; J15 3.9,0; J16 4.55,0; J17 5.2,0; K1 -5.2,-0.65; K1' 3.25,-0.65; K2 -4.55,-0.65; K3 -3.9,-0.65; K4 -3.25,-0.65; K15 3.9,-0.65; K16 4.55,-0.65; K17 5.2,-0.65; L1 -5.2,-1.3; L2 -4.55,-1.3; L3 -3.9,-1.3; L4 -3.25,-1.3; L14 3.25,-1.3; L15 3.9,-1.3; L16 4.55,-1.3; L17 5.2,-1.3; M1 -5.2,-1.95; M2 -4.55,-1.95; M3 -3.9,-1.95; M4 -3.25,-1.95; M14 3.25,-1.95; M16 4.55,-1.95; M17 5.2,-1.95; N1 -5.2,-2.6; N2 -4.55,-2.6; N3 -3.9,-2.6; N4 -3.25,-2.6; N14 3.25,-2.6; N15 3.9,-2.6; N16 4.55,-2.6; N17 5.2,-2.6; P1 -5.2,-3.25; P2 -4.55,-3.25; P3 -3.9,-3.25; P4 -3.25,-3.25; P5 -2.6,-3.25; P6 -1.95,-3.25; P7 -1.3,-3.25; P8 -0.65,-3.25; P9 0,-3.25; P10 0.65,-3.25; P11 1.3,-3.25; P12 1.95,-3.25; P13 2.6,-3.25; P14 3.25,-3.25; P15 3.9,-3.25; P16 4.55,-3.25; P17 5.2,-3.25; R1 -5.2,-3.9; R2 -4.55,-3.9; R3 -3.9,-3.9; R4 -3.25,-3.9; R5 -2.6,-3.9; R6 -1.95,-3.9; R7 -1.3,-3.9; R8 -0.65,-3.9; R9 0,-3.9; R10 0.65,-3.9; R11 1.3,-3.9; R12 1.95,-3.9; R13 2.6,-3.9; R14 3.25,-3.9; R15 3.9,-3.9; R16 4.55,-3.9; R17 5.2,-3.9; T1 -5.2,-4.55; T2 -4.55,-4.55; T3 -3.9,-4.55; T4 -3.25,-4.55; T5 -2.6,-4.55; T6 -1.95,-4.55; T7 -1.3,-4.55; T8 -0.65,-4.55; T9 0,-4.55; T10 0.65,-4.55; T11 1.3,-4.55; T12 1.95,-4.55; T13 2.6,-4.55; T14 3.25,-4.55; T15 3.9,-4.55; T16 4.55,-4.55; T17 5.2,-4.55; U1 -5.2,-5.2; U2 -4.55,-5.2; U3 -3.9,-5.2; U4 -3.25,-5.2; U5 -2.6,-5.2; U6 -1.95,-5.2; U7 -1.3,-5.2; U8 -0.65,-5.2; U9 0,-5.2; U10 0.65,-5.2; U11 1.3,-5.2; U12 1.95,-5.2; U13 2.6,-5.2; U14 3.25,-5.2; U15 3.9,-5.2; U16 4.55,-5.2; U17 5.2,-5.2
TMLF-6 = smd 0.25 x 0.7: 1 -0.5,-0.8; 2 0,-0.8; 3 0.5,-0.8; 4 0.5,0.8; 5 0,0.8; 6 -0.5,0.8 | smd 1.35 x 0.5: THERM 0,0
TO92 = drill 0.9 octagon: 1 -1.27,0; 2 0,1.905; 3 1.27,0
TO92-LINE = drill 0.9: 1 2.54,0; 2 0,0; 3 -2.54,0
TO252 = smd 1 x 1.6: 1 -2.28,-4.8; 2 2.28,-4.8 | smd 5.4 x 6.2: 3 0,2.5
TO263-5 = smd 1 x 3.4: 1 -3.4,-7.875; 2 -1.7,-7.875; 3 0,-7.875; 4 1.7,-7.875; 5 3.4,-7.875 | smd 10.414 x 9.525: 6 0,1.595
TO263-5_NOPASTE = smd 1 x 3.4: 1 -3.4,-9.145; 2 -1.7,-9.145; 3 0,-9.145; 4 1.7,-9.145; 5 3.4,-9.145 | smd 10.414 x 9.525: 6 0,0.325
TPS851 = smd 0.4 x 0.8: AOUT 0.65,-0.95; GND 0,0.95; NC1 -0.65,0.95; NC2 -0.65,-0.95; VCC 0.65,0.95
TPS61029 = smd 0.28 x 1.05: 1 -1,-1.6; 2 -0.5,-1.6; 3 0,-1.6; 4 0.5,-1.6; 5 1,-1.6; 6 1,1.6; 7 0.5,1.6; 8 0,1.6; 9 -0.5,1.6; 10 -1,1.6 | smd 2.4 x 1.6: GND1 0,0 | smd 0.8 x 0.28: GND2 -1.55,0.25; GND3 -1.55,-0.25; GND4 1.55,-0.25; GND5 1.55,0.25
TRIMPOT_BOURNS3MM = smd 1.2 x 1.2: A -1,-1.6; S 1,-1.6 | smd 1.6 x 1.5: E 0,1.65
TSL13T = smd 1.3 x 1: 1 -1.65,0.75; 2 -1.65,-0.75; 3 1.65,-0.75; 4 1.65,0.75
TSL2561_CS6 = smd 0.21 x 0.21: ADDR 0,-0.25; GND 0.5,-0.25; INT 0,0.25; SCL 0.5,0.25; SDA -0.5,0.25; VDD -0.5,-0.25
TSL2561_FN = smd 1.3 x 0.4: ADR -0.8,0; CLK 0.8,-0.65; DATA 0.8,0.65; INT 0.8,0; VDD -0.8,0.65; VSS -0.8,-0.65
TSOP54-400 = smd 0.4 x 0.9: 1 -10.4,-5.68; 2 -9.6,-5.68; 3 -8.8,-5.68; 4 -8,-5.68; 5 -7.2,-5.68; 6 -6.4,-5.68; 7 -5.6,-5.68; 8 -4.8,-5.68; 9 -4,-5.68; 10 -3.2,-5.68; 11 -2.4,-5.68; 12 -1.6,-5.68; 13 -0.8,-5.68; 14 0,-5.68; 15 0.8,-5.68; 16 1.6,-5.68; 17 2.4,-5.68; 18 3.2,-5.68; 19 4,-5.68; 20 4.8,-5.68; 21 5.6,-5.68; 22 6.4,-5.68; 23 7.2,-5.68; 24 8,-5.68; 25 8.8,-5.68; 26 9.6,-5.68; 27 10.4,-5.68; 28 10.4,5.68; 29 9.6,5.68; 30 8.8,5.68; 31 8,5.68; 32 7.2,5.68; 33 6.4,5.68; 34 5.6,5.68; 35 4.8,5.68; 36 4,5.68; 37 3.2,5.68; 38 2.4,5.68; 39 1.6,5.68; 40 0.8,5.68; 41 0,5.68; 42 -0.8,5.68; 43 -1.6,5.68; 44 -2.4,5.68; 45 -3.2,5.68; 46 -4,5.68; 47 -4.8,5.68; 48 -5.6,5.68; 49 -6.4,5.68; 50 -7.2,5.68; 51 -8,5.68; 52 -8.8,5.68; 53 -9.6,5.68; 54 -10.4,5.68 | smd 0.7 x 0.7: P$1 -11.75,-5.5
TSSOP5 = smd 0.35 x 0.55: 1 -0.65,-1.04; 2 0,-1.04; 3 0.65,-1.04; 4 0.65,0.95; 5 -0.65,0.94
TSSOP8 = smd 1.2 x 0.305: 1 -2.2,0.975; 2 -2.2,0.325; 3 -2.2,-0.325; 4 -2.2,-0.975; 5 2.2,-0.975; 6 2.2,-0.325; 7 2.2,0.325; 8 2.2,0.975
TSSOP8-4.4MM = smd 1.2 x 0.35: 1 -3.1,0.975; 2 -3.1,0.325; 3 -3.1,-0.325; 4 -3.1,-0.975; 5 3.1,-0.975; 6 3.1,-0.325; 7 3.1,0.325; 8 3.1,0.975
TSSOP14 = smd 0.305 x 0.991: 1 -1.95,-2.918; 2 -1.3,-2.918; 3 -0.65,-2.918; 4 0,-2.918; 5 0.65,-2.918; 6 1.3,-2.918; 7 1.95,-2.918; 8 1.95,2.918; 9 1.3,2.918; 10 0.65,2.918; 11 0,2.918; 12 -0.65,2.918; 13 -1.3,2.918; 14 -1.95,2.918
TSSOP16 = smd 0.305 x 0.991: 1 -2.275,-2.918; 2 -1.625,-2.918; 3 -0.975,-2.918; 4 -0.325,-2.918; 5 0.325,-2.918; 6 0.975,-2.918; 7 1.625,-2.918; 8 2.275,-2.918; 9 2.275,2.918; 10 1.625,2.918; 11 0.975,2.918; 12 0.325,2.918; 13 -0.325,2.918; 14 -0.975,2.918; 15 -1.625,2.918; 16 -2.275,2.918
TSSOP20 = smd 0.305 x 0.991: 1 -2.925,-2.918; 2 -2.275,-2.918; 3 -1.625,-2.918; 4 -0.975,-2.918; 5 -0.325,-2.918; 6 0.325,-2.918; 7 0.975,-2.918; 8 1.625,-2.918; 9 2.275,-2.918; 10 2.925,-2.918; 11 2.925,2.918; 12 2.275,2.918; 13 1.625,2.918; 14 0.975,2.918; 15 0.325,2.918; 16 -0.325,2.918; 17 -0.975,2.918; 18 -1.625,2.918; 19 -2.275,2.918; 20 -2.925,2.918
